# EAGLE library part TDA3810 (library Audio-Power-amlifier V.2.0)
The TDA3810 integrated circuit provides spatial, stereo and pseudo-stereo sound for radio and television equipment.
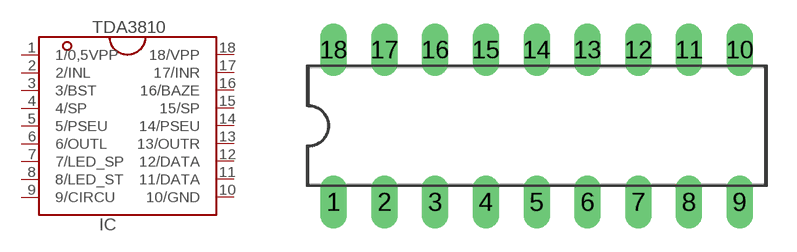
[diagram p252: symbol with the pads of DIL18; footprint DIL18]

Designator prefix IC

## TDA3810  [DIL18]
1  1/0,5VPP  pwr
2  2/INL  in
3  3/BST
4  4/SP
5  5/PSEU
6  6/OUTL  out
7  7/LED_SP  out
8  8/LED_ST  out
9  9/CIRCU
10  10/GND  pwr
11  11/DATA  in
12  12/DATA  in
13  13/OUTR  out
14  14/PSEU  in
15  15/SP
16  16/BAZE
17  17/INR  in
18  18/VPP  pwr

## Footprint DIL18 (pad centres in mm)
Dual In Line Package
drill 0.813 long: 1 -10.16,-3.81; 2 -7.62,-3.81; 3 -5.08,-3.81; 4 -2.54,-3.81; 5 0,-3.81; 6 2.54,-3.81; 7 5.08,-3.81; 8 7.62,-3.81; 9 10.16,-3.81; 10 10.16,3.81; 11 7.62,3.81; 12 5.08,3.81; 13 2.54,3.81; 14 0,3.81; 15 -2.54,3.81; 16 -5.08,3.81; 17 -7.62,3.81; 18 -10.16,3.81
